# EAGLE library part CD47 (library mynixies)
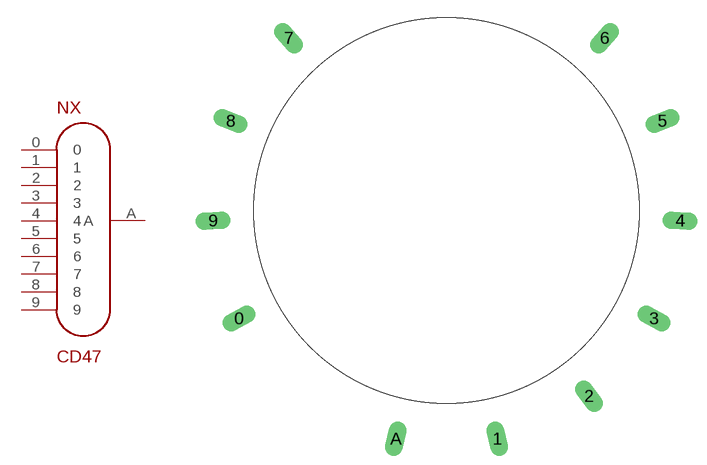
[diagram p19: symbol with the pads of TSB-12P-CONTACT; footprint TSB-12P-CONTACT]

Designator prefix NX

## CD47  [TSB-12P-CONTACT]
0  0  pas
1  1  pas
2  2  pas
3  3  pas
4  4  pas
5  5  pas
6  6  pas
7  7  pas
8  8  pas
9  9  pas
A  A  pas

## Footprint TSB-12P-CONTACT (pad centres in mm)
drill 1 long: 0 -17.74,-9.235; 1 4.329,-19.526; 2 12.175,-15.867; 3 17.74,-9.235; 4 19.981,-0.872; 5 18.478,7.654; 6 13.512,14.746; 7 -13.512,14.746; 8 -18.478,7.654; 9 -19.981,-0.872; A -4.329,-19.526
hole 33 at 0,0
